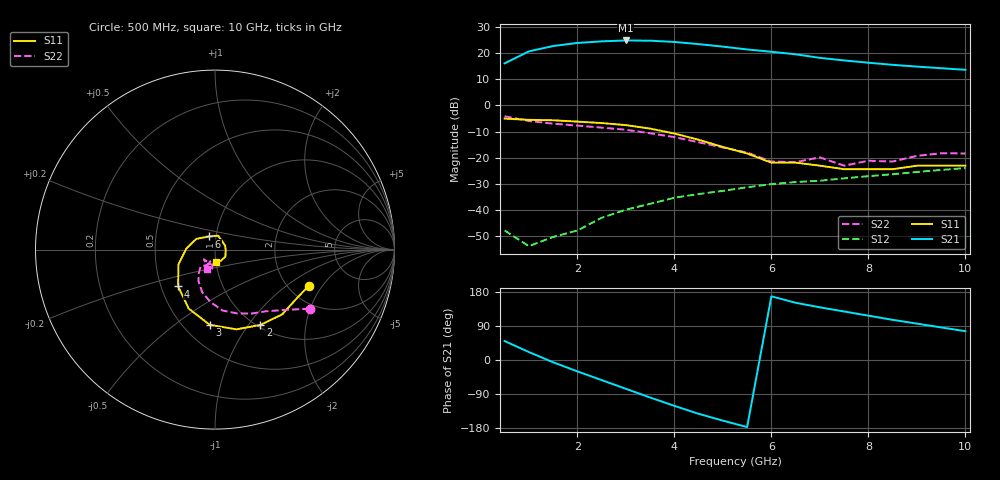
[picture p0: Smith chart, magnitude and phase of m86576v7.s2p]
!MGA-86576 S PARAMETERS
!Vd=7V LAST UPDATED 07-01-94
# ghz s ma r 50
!FREQ  S11  S21  S12  S22
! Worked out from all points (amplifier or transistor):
!   20 points, 500 MHz to 10 GHz, reference 50 ohm
!   highest |S21| = 24.9 dB at 3 GHz (marker M1)
!   |S21| within 3 dB of that: 1.29 GHz to 5.292 GHz (4.002 GHz wide, 122 % of centre)
!   unconditionally stable (mu >= 1): start of sweep to end of sweep
!   at 2 GHz: K = 5.22, MAG = 25.8 dB, |S12| = -48.0 dB
!   at 5.5 GHz: K = 1.68, MAG = 21.6 dB, |S12| = -31.4 dB
!   at 10 GHz: K = 1.75, MAG = 13.8 dB, |S12| = -24.0 dB
!   S11 on the Smith chart (normalised r, x): 500 MHz: 2.56, -1.50; 2 GHz: 1.03, -1.14; 3 GHz: 0.67, -0.68; 4 GHz: 0.61, -0.27; 6 GHz: 0.93, +0.14; 10 GHz: 1.00, -0.14
0.5  0.56 -21.0  6.42 50.0  0.004 -15.0  0.621 -32.0
1  0.53 -31.0  10.91 21.0  0.002 17.0  0.504 -42.0
1.5  0.52 -44.0  13.81 -6.0  0.003 62.0  0.448 -50.0
2  0.49 -59.0  15.83 -30.0  0.004 85.0  0.411 -60.0
2.5  0.46 -75.0  16.99 -53.0  0.007 96.0  0.376 -71.0
3  0.42 -94.0  17.67 -76.0  0.01 98.0  0.342 -83.0
3.5  0.36 -114.0  17.48 -99.0  0.013 97.0  0.293 -95.0
4  0.29 -135.0  16.55 -121.0  0.017 94.0  0.247 -107.0
4.5  0.22 -158.0  15.03 -142.0  0.02 91.0  0.197 -118.0
5  0.16 178.0  13.45 -160.0  0.023 88.0  0.156 -125.0
5.5  0.12 150.0  11.88 -177.0  0.027 85.0  0.125 -130.0
6  0.08 114.0  10.72 168.0  0.031 83.0  0.084 -110.0
6.5  0.08 77.0  9.58 151.0  0.034 77.0  0.082 -139.0
7  0.07 68.0  8.19 139.0  0.036 75.0  0.101 -116.0
7.5  0.06 42.0  7.31 128.0  0.04 73.0  0.07 -112.0
8  0.06 21.0  6.61 117.0  0.044 71.0  0.087 -109.0
8.5  0.06 -3.0  6.02 106.0  0.048 69.0  0.084 -99.0
9  0.07 -34.0  5.57 96.0  0.053 66.0  0.108 -99.0
9.5  0.07 -62.0  5.18 86.0  0.058 63.0  0.121 -105.0
10  0.07 -84.0  4.84 76.0  0.063 59.0  0.12 -113.0
